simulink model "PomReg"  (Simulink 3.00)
settings: Solver=ode45  StartTime=0.0  StopTime=10.0  RelTol=1e-3
libraries: simulink_extras x1

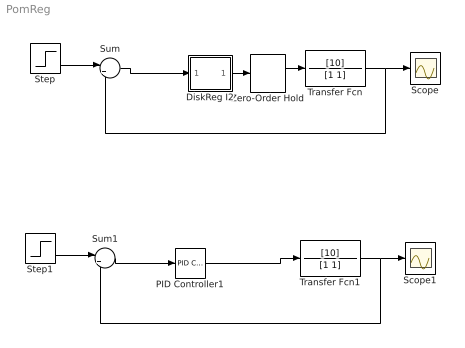
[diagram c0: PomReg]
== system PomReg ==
  DiskReg I2 : Subsystem
  PID Controller1 : simulink_extras/Additional Linear/PID Controller  P=1/10  I=0.1  D=0
  Scope : Scope
  Scope1 : Scope
  Step : Step  Time=0  Before=0  After=1  SampleTime=0
  Step1 : Step  Time=0  Before=0  After=1  SampleTime=0
  Sum : Sum  Inputs=|+-  SaturateOnIntegerOverflow=on
  Sum1 : Sum  Inputs=|+-  SaturateOnIntegerOverflow=on
  Transfer Fcn : TransferFcn  Numerator=[10]  Denominator=[1 1]
  Transfer Fcn1 : TransferFcn  Numerator=[10]  Denominator=[1 1]
  Zero-Order Hold : ZeroOrderHold  SampleTime=0.01
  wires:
  Step/1 -> Sum/1
  Transfer Fcn/1 -> Scope/1, Sum/2
  DiskReg I2/1(Out1) -> Zero-Order Hold/1
  Zero-Order Hold/1 -> Transfer Fcn/1
  Sum/1 -> DiskReg I2/1(In1)
  Step1/1 -> Sum1/1
  Transfer Fcn1/1 -> Sum1/2, Scope1/1
  Sum1/1 -> PID Controller1/1
  PID Controller1/1 -> Transfer Fcn1/1

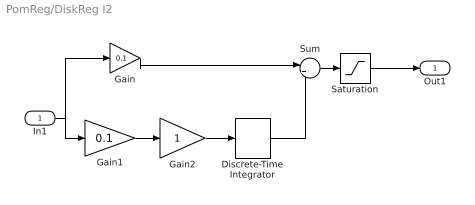
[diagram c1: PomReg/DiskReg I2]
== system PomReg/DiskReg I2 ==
  In1 : Inport  Port=1  PortWidth=-1  SampleTime=-1  DataType=auto
  Discrete-Time Integrator : DiscreteIntegrator  IntegratorMethod=ForwardEuler  ExternalReset=none  InitialConditionSource=internal  InitialCondition=0  LimitOutput=off  UpperSaturationLimit=inf  LowerSaturationLimit=-inf  ShowSaturationPort=off  ShowStatePort=off  SampleTime=0.01
  Gain : Gain  Gain=0.1  SaturateOnIntegerOverflow=on
  Gain1 : Gain  Gain=0.1  SaturateOnIntegerOverflow=on
  Gain2 : Gain  Gain=1  SaturateOnIntegerOverflow=on
  Saturation : Saturate  UpperLimit=311  LowerLimit=-311
  Sum : Sum  Inputs=|++  SaturateOnIntegerOverflow=on
  Out1 : Outport  Port=1
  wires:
  In1/1 -> Gain/1, Gain1/1
  Discrete-Time Integrator/1 -> Sum/2
  Gain/1 -> Sum/1
  Gain2/1 -> Discrete-Time Integrator/1
  Gain1/1 -> Gain2/1
  Sum/1 -> Saturation/1
  Saturation/1 -> Out1/1
